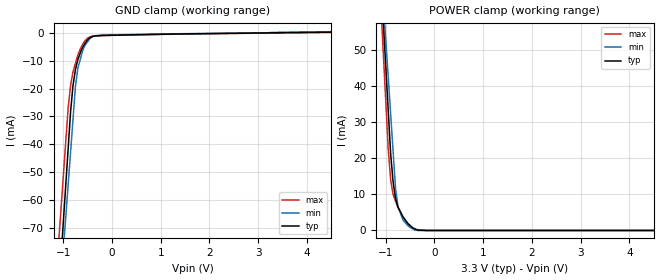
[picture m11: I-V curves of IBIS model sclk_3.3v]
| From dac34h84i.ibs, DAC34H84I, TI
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[Model] sclk_3.3v
Model_type Input
Vinl = 990.000mV
Vinh = 2.31000V
C_comp 641.000fF 640.000fF 642.000fF
| variable typ   min   max
[Voltage Range] 3.30000V 3.00000V 3.60000V
[POWER Clamp Reference] 3.30000V 3.00000V 3.60000V
[GND Clamp Reference] 0.00000V 0.00000V 0.00000V
[Temperature Range] 25   125   -40
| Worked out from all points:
|   GND clamp passes 1 mA (typ) near -0.28 V on its own axis
|   POWER clamp passes 1 mA (typ) near -0.47 V on its own axis
[GND Clamp]
-3.3V     -680.9mA   -621.5mA   -621mA
-900mV    -41.6mA    -54.6mA    -26.94mA
-850mV    -28.28mA   -42.79mA   -18.79mA
-800mV    -18.83mA   -30.98mA   -13.91mA
-750mV    -13.08mA   -19.17mA   -10.86mA
-700mV    -9.489mA   -12.61mA   -7.806mA
-600mV    -5.039mA   -6.221mA   -3.959mA
-550mV    -3.717mA   -4.31mA    -2.679mA
-450mV    -1.682mA   -1.988mA   -1.39mA
-350mV    -1.064mA   -1.03mA    -1.104mA
-175mV    -899.8uA   -751.7uA   -949uA
6.6V      731.5uA    873.6uA    588.4uA
[POWER Clamp]
-3.3V     600.5mA    526.6mA    642.1mA
-1.15V    81.6mA     83.79mA    75.3mA
-1.05V    57.47mA    63.19mA    48.94mA
-950mV    33.34mA    42.6mA     22.58mA
-900mV    21.27mA    32.3mA     14.01mA
-850mV    13.49mA    22.01mA    9.972mA
-800mV    8.806mA    11.71mA    8.17mA
-750mV    6.482mA    6.74mA     6.368mA
-650mV    3.848mA    2.967mA    3.762mA
-550mV    1.997mA    1.352mA    1.875mA
-400mV    453.6uA    135.2uA    225uA
6.6V      0A         0A         0A
